VAR_GLOBAL CONSTANT
	cTaskCycleTime	: LREAL 	:= 1.0; 									// Cycle time of sampling task in ms.
	cOversamples 	: UDINT 	:= 10;										// Number of oversamples
	cSampleRate		: LREAL		:= 1E3 * cOversamples / cTaskCycleTime;		// Sample rate of input signal.
	
	cBufferLength	: UDINT		:= 1024;									// Buffer size
	cWindowLength	: UDINT		:= 2048;									// Internal buffer size with 50% overlapping
	
	cResolution		: LREAL 	:= cSamplerate / cWindowLength;				// Frequency resolution
	cBands			: UDINT 	:= 2;										// Number of bands
	cSetFrequency	: ARRAY[1..cBands] OF LREAL := [ 41*cResolution, 413 ];	// Frequency in Hz; [ exact, intermediate ]
	cSetAmplitude	: ARRAY[1..cBands] OF LREAL := [ 1.0, 2.0 ];			// Peak amplitudes of sine signals
	
	cBandWidth		: UDINT		:= 5;										// Computed bins per frequency.
	cDFTBins		: UDINT		:= cBandWidth * cBands;						// Number of spectral bins, cBandWidth bins per frequency
	
END_VAR
